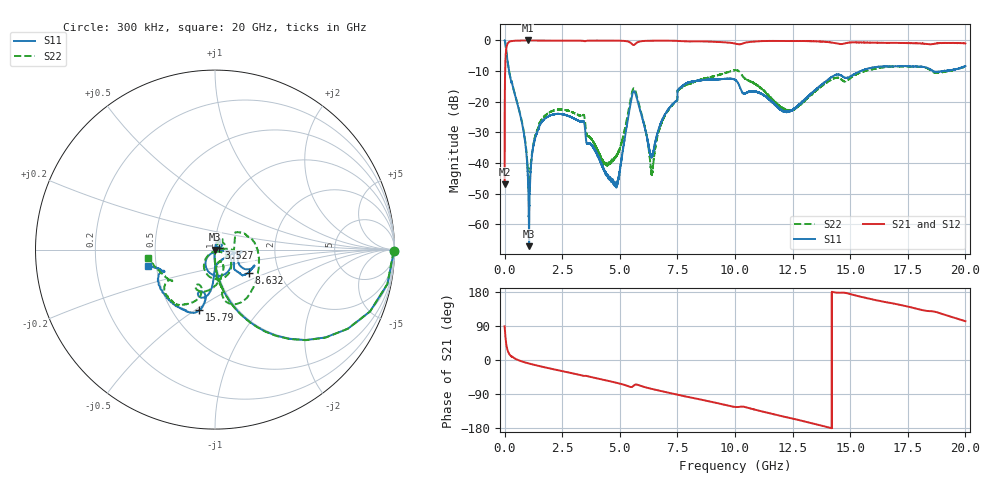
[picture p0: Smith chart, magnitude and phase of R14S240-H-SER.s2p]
!{R14S240}
!Johanson Technology Inc.
!www.johansontechnology.com
!Test Board Conditions:
!Substrate Type  RO4350B
!Substrate Thickness  20 mil
!Substrate Dk  3.66
!TL Type: GCPW
!TL Trace Width  36 mil
!TL Gap  12 mil
!Electrode orientation  Horizontal
!DUT TOPOLOGY	SERIES
!Mounting Pad LxW  26x36 mil
! Created Wed Nov 25 17:33:21 2020
! 2 Port Network Data from SP1.SP block
! freq  magS11  angS11  magS21  angS21  magS12  angS12  magS22  angS22
# khz S ma R 50
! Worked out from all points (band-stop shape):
!   20001 points, 300 kHz to 20 GHz, reference 50 ohm
!   highest |S21| = -0.01 dB at 994.3 MHz (marker M1); lowest = -46.9 dB at 300 kHz (marker M2)
!   |S21| within 3 dB of the highest: 67.09 MHz to end of sweep
!   lowest |S11| = -67.1 dB at 1.064 GHz (marker M3), VSWR 1.00, Z = 50 + j0.0271 ohm
!   |S11| at or under -10 dB: 193.9 MHz to 15.46 GHz (15.27 GHz wide, 195 % of centre); 18.61 GHz to 19.01 GHz (395.3 MHz wide, 2.1 % of centre); 19.03759 GHz to 19.04692 GHz (9.325 MHz wide, 0.049 % of centre)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
!   |S22| runs from -49.6 to 0.0 dB; largest |S21 - S12| = 0.021
!   S11 on the Smith chart (normalised r, x): 300 kHz: open; 3.527 GHz: 1.05, +0.02; 8.632 GHz: 1.40, -0.38; 15.79 GHz: 0.68, -0.52; 20 GHz: 0.45, -0.10
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300  0.9972 -0.3  0.004499 89.0  0.004457 88.6  0.9952 -0.5
140300  0.4232 -65.9  0.9019 23.9  0.9039 23.8  0.4253 -65.9
802300  0.03627 -93.9  0.9979 -4.8  0.9969 -4.8  0.03817 -91.0
994300  0.008054 -102.1  0.9991 -8.2  0.9981 -8.2  0.00948 -80.8
1064300  0.0004406 142.0  0.9978 -9.3  0.9971 -9.3  0.00376 -11.9
1284300  0.02212 81.4  0.9979 -12.8  0.9977 -12.7  0.02343 65.6
1637300  0.04774 72.3  0.9961 -17.9  0.9962 -17.9  0.05257 69.8
3334300  0.04745 52.6  0.9908 -40.5  0.9916 -40.4  0.0594 41.1
3527300  0.02539 24.4  0.9789 -41.8  0.9792 -41.8  0.03534 7.7
4344300  0.007272 94.2  0.996 -53.0  0.995 -53.0  0.009862 -23.6
4808300  0.004528 97.4  0.9927 -59.4  0.9926 -59.4  0.01245 -53.6
5592300  0.1471 -67.5  0.8413 -68.4  0.8416 -68.4  0.1647 -74.2
6370300  0.01258 -76.9  0.99 -76.0  0.9894 -76.0  0.007068 -88.2
6667300  0.03386 -12.2  0.9904 -80.2  0.9905 -80.2  0.0304 4.2
7600300  0.1671 -45.1  0.9775 -92.9  0.9782 -92.8  0.1615 36.5
8632300  0.2271 -34.3  0.9644 -106.0  0.9634 -105.9  0.2374 0.1
1.00003e7  0.2281 -27.4  0.8904 -124.0  0.8887 -123.9  0.3274 -61.8
1.22633e7  0.06843 -59.1  0.9804 -151.4  0.9815 -151.3  0.0731 -72.6
1.33343e7  0.139 -92.0  0.9721 -166.7  0.9745 -166.7  0.1319 -70.5
1.57893e7  0.3486 -104.5  0.9195 162.4  0.9232 162.3  0.3273 -114.5
1.66673e7  0.3747 -115.8  0.9139 151.4  0.9047 151.1  0.3738 -123.8
2e7  0.3815 -166.3  0.8964 102.4  0.896 102.9  0.376 -172.8
